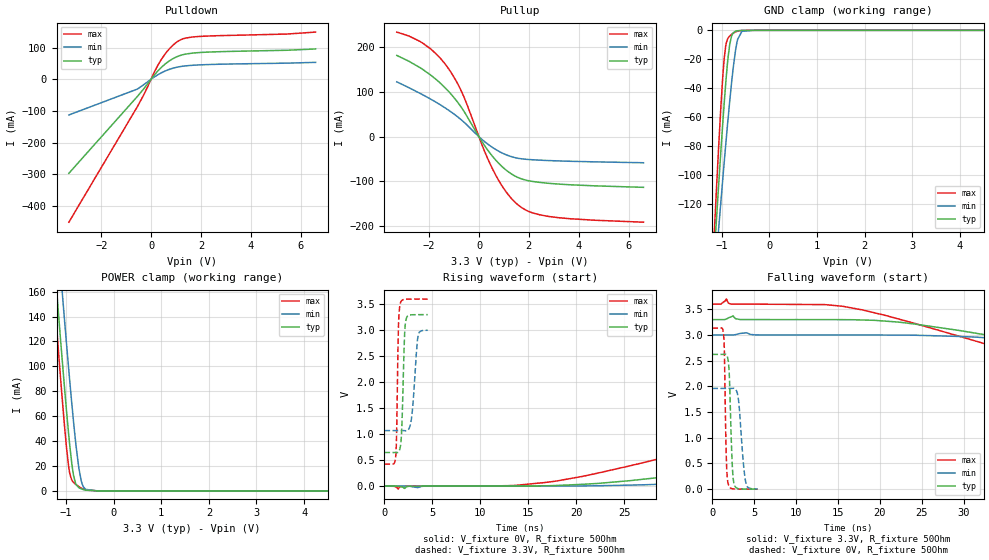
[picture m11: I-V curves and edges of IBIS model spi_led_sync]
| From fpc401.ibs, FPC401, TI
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|   spi_led_sync Model
[Model]   spi_led_sync
Model_type   I/O
Polarity   Non-Inverting
Enable   Active-Low
Vinl = 0.8
Vinh = 2.0
Vmeas = 1.65
Vref = 3.3
Cref = 200pF
Rref = 50
|   typ   min   max
C_comp   5.269e-10   3.345e-10   6.900e-10
| Where nom  PVT is Nominal Process, 3.3V, 27C
|   Fast PVT is Strong Process,  3.6V, -40C
|   Slow PVT is Weak Process,   3V, 125C
[Voltage Range]   3.3   3   3.6
|Junction Temperature
[Temperature Range]   27   125   -40
[Pullup Reference]   3.3   3   3.6
[Pulldown Reference]   0   0   0
[Power Clamp Reference]   3.3   3   3.6
[GND Clamp Reference]   0   0   0
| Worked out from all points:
|   slope of the pulldown table from 0 to 0.495 V, typ, clamps not added: 11.5 ohm
|   slope of the pullup table from 0 to 0.495 V, typ, clamps not added: 12.3 ohm
|   GND clamp passes 1 mA (typ) near -0.73 V on its own axis
|   POWER clamp passes 1 mA (typ) near -0.63 V on its own axis
|   falling waveform, V_fixture 3.3V, R_fixture 50Ohm: 20-80 % time 72ns typ, 116ns min, 46.6ns max; typ from 3.3 V to 0.647 V
|   rising waveform, V_fixture 0V, R_fixture 50Ohm: 20-80 % time 66.8ns typ, 113ns min, 41.5ns max; typ from 0 V to 2.62 V
|   rising waveform, V_fixture 3.3V, R_fixture 50Ohm: 20-80 % time 251ps typ, 441ps min, 173ps max; typ from 0.646 V to 3.3 V
|   falling waveform, V_fixture 0V, R_fixture 50Ohm: 20-80 % time 311ps typ, 552ps min, 208ps max; typ from 2.62 V to 0.001 V
[Pulldown]
|   Voltage   I(typ)   I(min)   I(max)
-3.3V     -296.2mA   -112.4mA   -450.4mA
-549mV    -53.89mA   -30.73mA   -85.92mA
-153.6mV  -15.8mA    -8.74mA    -26.02mA
153mV     15.81mA    8.562mA    26.43mA
381mV     35.36mA    19.17mA    58.75mA
702mV     56.43mA    30.51mA    93.34mA
1.035V    71.18mA    38.14mA    117.6mA
1.344V    78.94mA    42.03mA    129.2mA
1.848V    83.87mA    45.07mA    134.6mA
5.441V    91.55mA    50.91mA    142.7mA
6.6V      95.65mA    53.4mA     148.8mA
[GND Clamp]
|   Voltage   I(typ)   I(min)   I(max)
-3.3V     -1.371A    -1.102A    -1.688A
-1.197V   -174.4mA   -189.4mA   -164.6mA
-1.111V   -129mA     -154.3mA   -107.7mA
-1.073V   -109mA     -138.6mA   -83.2mA
-1.021V   -83.21mA   -118.2mA   -52.74mA
-948mV    -48.8mA    -89.75mA   -18.42mA
-906mV    -31.32mA   -73.97mA   -8.542mA
-834.9mV  -9.545mA   -48.67mA   -3.877mA
-717mV    -692.6uA   -14.58mA   -1.187mA
-579mV    -49.3uA    -678.8uA   -97.43uA
-330mV    -89.4nA    -746.6nA   -56.52nA
6.6V      0A         0A         0A
[Pullup]
|   Voltage   I(typ)   I(min)   I(max)
-3.3V     182mA      123mA      234.3mA
-2.244V   150.2mA    93.52mA    209mA
-1.734V   128.8mA    77.57mA    186.2mA
-1.211V   100.9mA    59mA       151.4mA
-620.4mV  58.34mA    33.49mA    91.03mA
165mV     -14.93mA   -8.222mA   -24.57mA
660mV     -51.63mA   -28.25mA   -84.9mA
1.15V     -77.44mA   -41.75mA   -128.1mA
1.647V    -93.19mA   -48.99mA   -156.2mA
2.143V    -100mA     -51.54mA   -170.4mA
2.832V    -104.4mA   -53.42mA   -178.7mA
6.6V      -113.3mA   -58.24mA   -191.3mA
[POWER Clamp]
|   Voltage   I(typ)   I(min)   I(max)
-3.3V     1.286A     1.299A     1.304A
-1.295V   209.4mA    262.1mA    181.2mA
-1.158V   141.9mA    196.1mA    111.5mA
-1.098V   113.3mA    167.8mA    82.31mA
-1.036V   84.38mA    138.8mA    53.6mA
-916.8mV  34.69mA    85.98mA    13.16mA
-858mV    16.09mA    61.61mA    7.537mA
-801.9mV  6.242mA    40.33mA    5.442mA
-684mV    1.719mA    8.545mA    2.353mA
-588mV    607.1uA    1.225mA    772.7uA
-330mV    2.194uA    7.268uA    1.05uA
6.6V      0A         0A         0A
[Ramp]
R_load = 50
|   typ   min   max
dV/dt_r   1.574/6.68506e-08   1.17602/1.13628e-07   1.8813/4.14828e-08
dV/dt_f   1.59231/7.15637e-08   1.15919/1.16555e-07   1.90616/4.65999e-08
[Falling Waveform]
V_fixture = 3.3V
V_fixture_min = 3V
V_fixture_max = 3.6V
R_fixture = 50Ohm
|   Time   V(typ)   V(min)   V(max)
0s        3.3V       3V         3.6V
1.661ns   3.311V     3V         3.7V
17.93ns   3.292V     3V         3.488V
31.51ns   3.033V     2.959V     2.878V
54.71ns   2.375V     2.638V     1.827V
77.72ns   1.798V     2.303V     1.018V
108.1ns   1.235V     1.941V     622.3mV
151.3ns   869.2mV    1.578V     498mV
248.3ns   694.5mV    1.219V     437.8mV
608.3ns   646.7mV    1.071V     423.2mV
[Rising Waveform]
V_fixture = 0V
V_fixture_min = 0V
V_fixture_max = 0V
R_fixture = 50Ohm
|   Time   V(typ)   V(min)   V(max)
0s        445.8pV    23.55nV    91.52pV
13.46ns   -175.4uV   -499.5uV   10.46mV
20.69ns   34.54mV    3.106mV    188.4mV
58.59ns   952.9mV    382.3mV    1.981V
72.32ns   1.318V     569.6mV    2.512V
100ns     1.938V     924.2mV    2.89V
136.6ns   2.331V     1.299V     3.018V
188.3ns   2.49V      1.648V     3.084V
228.3ns   2.543V     1.772V     3.106V
608.3ns   2.622V     1.955V     3.135V
[Rising Waveform]
V_fixture = 3.3V
V_fixture_min = 3V
V_fixture_max = 3.6V
R_fixture = 50Ohm
|   Time   V(typ)   V(min)   V(max)
0s        646.2mV    1.068V     423.1mV
1.17ns    646.3mV    1.068V     565.5mV
1.279ns   645.4mV    1.068V     1.113V
1.462ns   656.5mV    1.068V     3.082V
1.661ns   763mV      1.068V     3.52V
1.79ns    1.044V     1.068V     3.569V
2.209ns   3.169V     1.065V     3.595V
2.841ns   3.296V     1.335V     3.598V
3.535ns   3.299V     2.925V     3.599V
4.51ns    3.299V     2.999V     3.599V
[Falling Waveform]
V_fixture = 0V
V_fixture_min = 0V
V_fixture_max = 0V
R_fixture = 50Ohm
|   Time   V(typ)   V(min)   V(max)
0s        2.623V     1.96V      3.136V
1.316ns   2.623V     1.96V      3.043V
1.426ns   2.624V     1.96V      2.737V
1.661ns   2.618V     1.96V      634.6mV
1.906ns   2.48V      1.96V      93.85mV
2.327ns   652.5mV    1.961V     10.42mV
2.571ns   109.1mV    1.963V     4.111mV
3.118ns   8.238mV    1.74V      1.448mV
4.05ns    434.9uV    92.25mV    262.8uV
5.418ns   771.5uV    1.336mV    320.9uV
